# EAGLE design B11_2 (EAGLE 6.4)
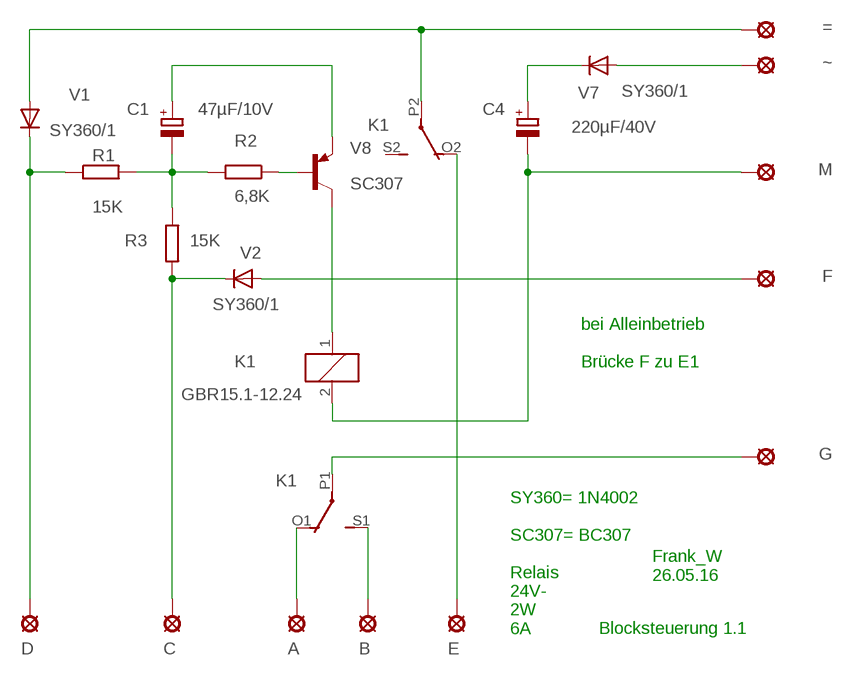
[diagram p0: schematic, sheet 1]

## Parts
=  LSP10  [LSP10]
A  LSP10  [LSP10]
B  LSP10  [LSP10]
C  LSP10  [LSP10]
C1  47µF/10V  CPOL-EUE5-5  [E5-5]
C4  220µF/40V  CPOL-EUE22-9AXIAL  [E22-9]
D  LSP10  [LSP10]
E  LSP10  [LSP10]
F  LSP10  [LSP10]
G  LSP10  [LSP10]
K1  GBR15.1-12.24  4052  [F4052]
M  LSP10  [LSP10]
R1  15K  R-EU_0207/12  [0207/12]
R2  6,8K  R-EU_0207/12  [0207/12]
R3  15K  R-EU_0207/12  [0207/12]
V1  SY360/1  1N4004  [DO41-10]
V2  SY360/1  1N4004  [DO41-10]
V7  SY360/1  1N4004  [DO41-10]
V8  SC307  BC307  [TO92]
~  LSP10  [LSP10]

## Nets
N$1: F.MP V2.A
N$2: C4.- K1.2 M.MP
N$3: =.MP K1.P2(3:P) V1.A
N$4: C4.+ V7.C
N$5: K1.1 V8.3(C)
N$6: C1.- R1.2 R2.2 R3.1
N$7: A.MP K1.O1(2:O)
N$8: R2.1 V8.2(B)
N$9: D.MP R1.1 V1.C
N$10: C.MP R3.2 V2.C
N$12: B.MP K1.S1(2:S)
N$13: V7.A ~.MP
N$14: E.MP K1.O2(3:O)
N$25: G.MP K1.P1(2:P)
N$42: C1.+ V8.1(E)
Unconnected: K1.S2(3:S)

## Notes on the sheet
- bei Alleinbetrieb
  
  Brücke F zu E1
- Frank_W 
  26.05.16
- SY360= 1N4002 
  
  SC307= BC307
  
  Relais 
  24V-
  2W
  6A
- Blocksteuerung 1.1

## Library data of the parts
= A B C D E F G M ~ = solpad:LSP10: SOLDER PAD
C1 C4 = rcl:CPOL-EU: POLARIZED CAPACITOR, European symbol
K1 = relay:4052: RELAY 2 x switch, Finder; OC_FARNELL: unknown; OC_NEWARK: unknown
R1-R3 = rcl:R-EU_: RESISTOR, European symbol
V1 V2 V7 = diode:1N4004: DIODE
V8 = transistor-pnp:BC307: PNP Transistor

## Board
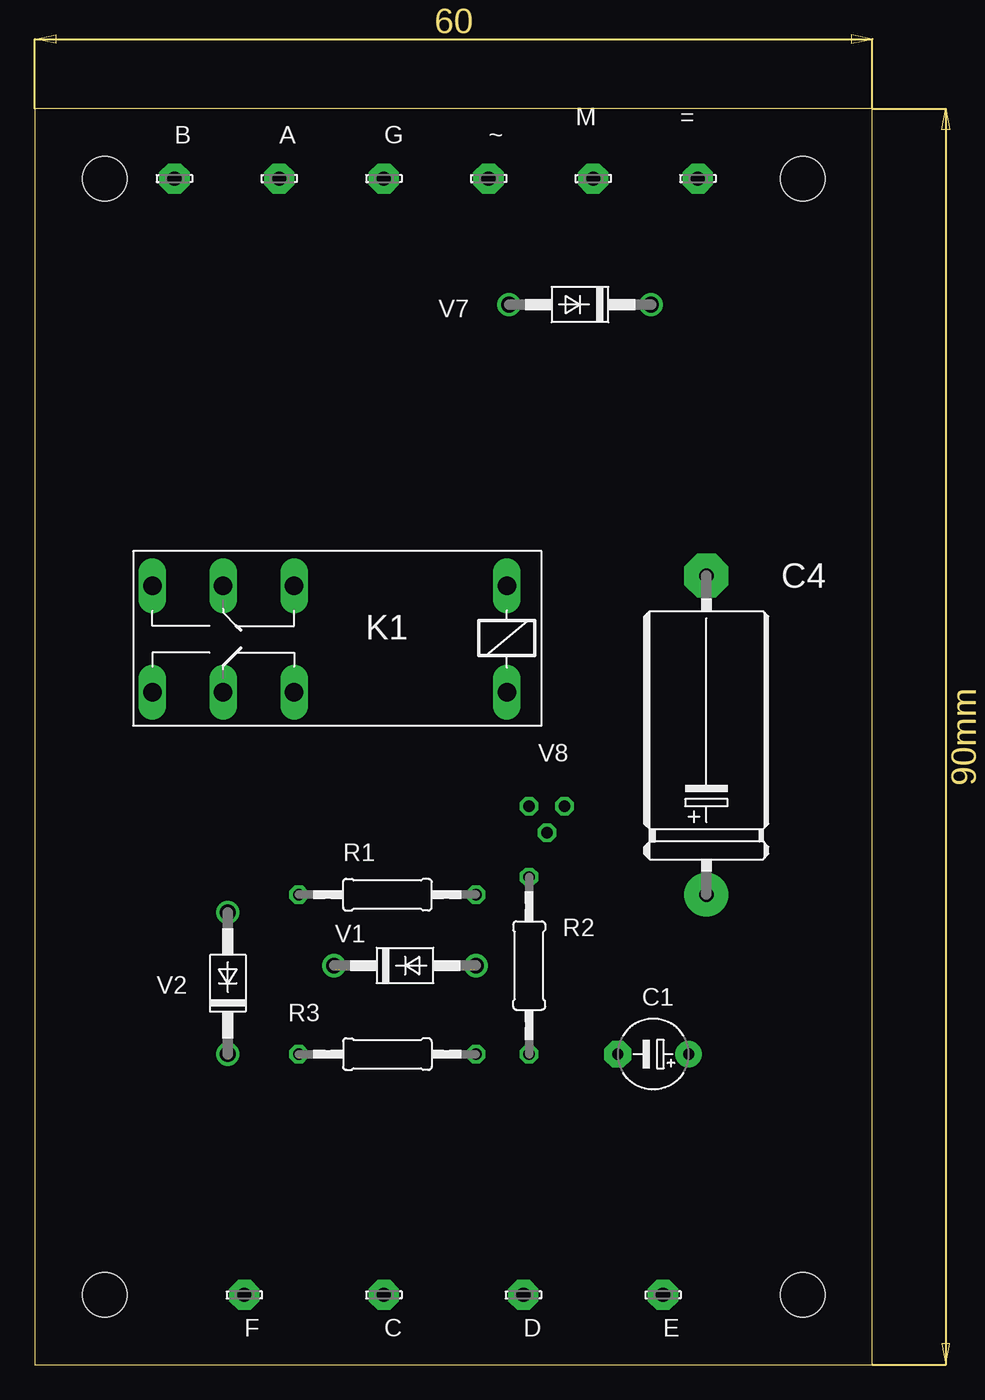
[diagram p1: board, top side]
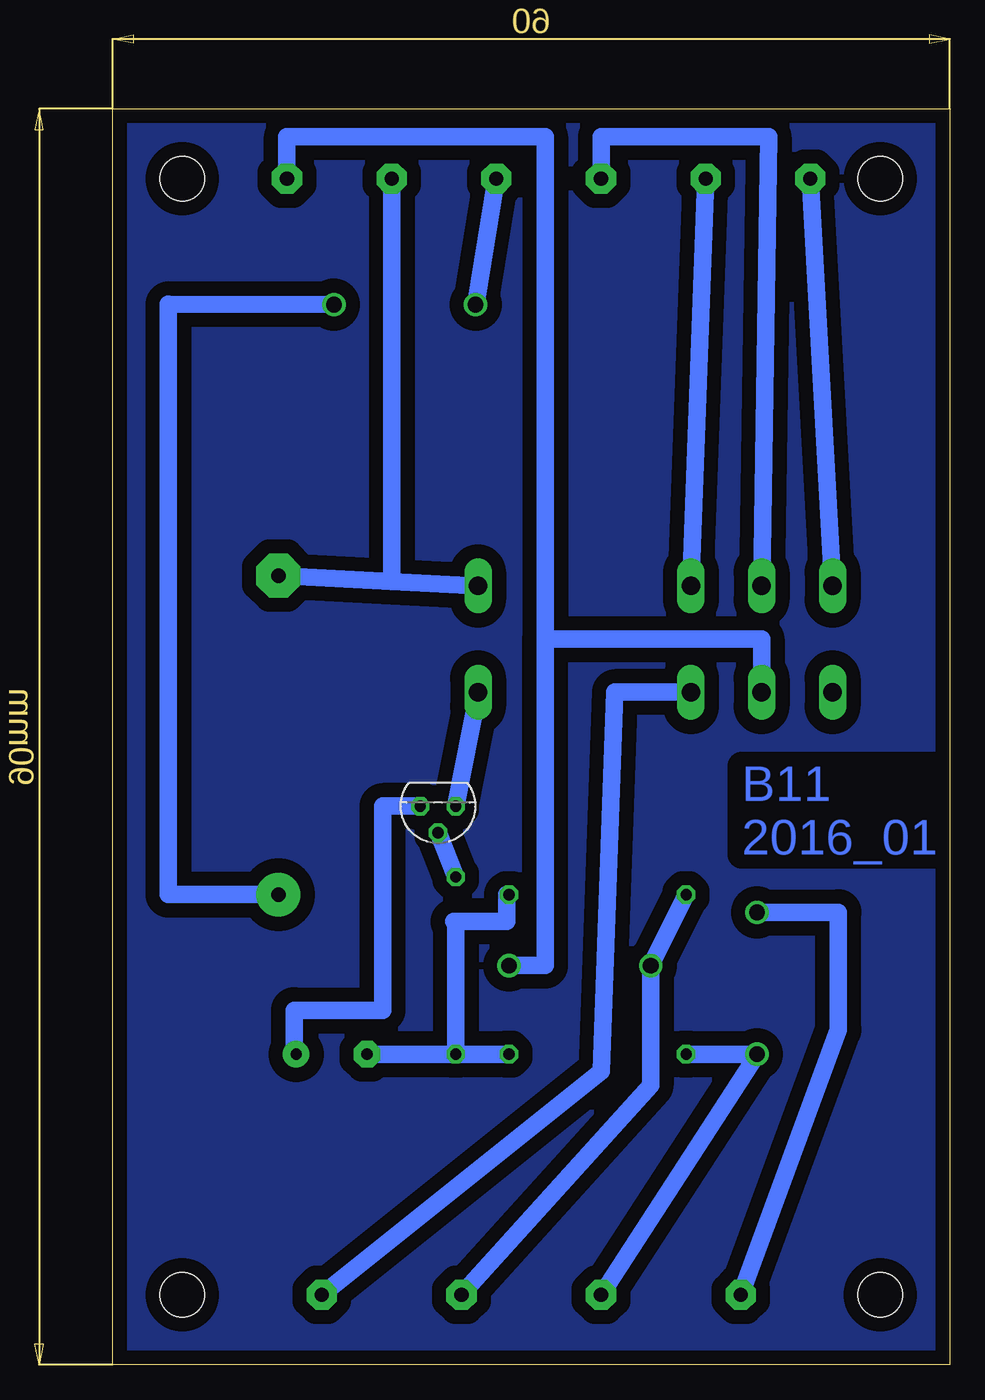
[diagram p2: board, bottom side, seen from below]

Size 65.56 x 95.3 mm. Coordinates in mm from the lower left corner, seen from the top.
Outline: 0,90 0,0 60,0 60,90 0,90
Copper layers (1*16): Top 0.035mm / dielectric 1.5mm / Bottom 0.035mm
Design rules "default *": minimum track width 20mil, minimum drill 24mil, track to track 8mil, track to pad 8mil, pad to pad 8mil, via to via 8mil, smd to smd 8mil, copper to edge 40mil, drill to drill 8mil, minimum pad ring 10mil, minimum via ring 8mil, stop-mask expansion 4mil, vias tented up to drill 0mil, thermal gap 20mil
Holes 3.2 mm at 55,5 5,85 5,5 55,85

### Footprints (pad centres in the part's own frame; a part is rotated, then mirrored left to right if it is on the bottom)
LSP10 = drill 1.016 pad 2.159 octagon: MP 0,0
E5-5 = drill 0.813 pad 1.905: + -2.54,0 | drill 0.813 pad 1.905 octagon: - 2.54,0
E22-9 = drill 1.016 pad 3.15: + -11.43,0 | drill 1.016 pad 3.15 octagon: - 11.43,0
F4052 = drill 1.321 long: 1 -3.81,3.81; 2 -3.81,-3.81; O1 11.43,-3.81; O2 11.43,3.81; P1 16.51,-3.81; P2 16.51,3.81; S1 21.59,-3.81; S2 21.59,3.81
0207/12 = drill 0.813 octagon: 1 -6.35,0; 2 6.35,0
DO41-10 = drill 1.118: A 5.08,0; C -5.08,0
TO92 = drill 0.813 octagon: 1 1.27,0; 2 0,1.905; 3 -1.27,0

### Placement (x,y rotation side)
=  47.5,85 0 top
A  17.5,85 0 top
B  10,85 0 top
C  25,5 0 top
C1  44.3,22.25 180 top
C4  48.11,45.11 90 top
D  35,5 0 top
E  45,5 0 top
F  15,5 0 top
G  25,85 0 top
K1  30,52 180 top
M  40,85 0 top
R1  25.25,33.68 0 top
R2  35.41,28.6 270 top
R3  25.25,22.25 180 top
V1  26.52,28.6 0 top
V2  13.82,27.33 90 top
V7  39.06,75.97 180 top
V8  36.68,40.03 180 bottom
~  32.5,85 0 top

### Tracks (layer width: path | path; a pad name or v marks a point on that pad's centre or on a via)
N$1
  Bottom 1.27: F.MP 8,24 8,32.41 V2.A
N$2
  Bottom 1.27: C4.- 39.99,56.13 | 39.99,56.13 K1.2 | M.MP 39.99,56.13
N$3
  Bottom 1.27: =.MP 47.5,88 29,88 29,52 | 29,52 13.49,52 K1.P2 | V1.A 29,28.6 29,52
N$4
  Bottom 1.27: V7.C 56,76 56,33.68 C4.+
N$5
  Bottom 1.27: V8.3 K1.1
N$6
  Bottom 1.27: R3.1 R2.2 | R2.2 C1.- | R1.2 31.75,33.68 31.75,31.75 35.41,31.75 | 35.56,31.75 35.41,31.75 | 35.41,31.75 R2.2
N$7
  Bottom 1.27: K1.O1 A.MP
N$8
  Bottom 1.27: R2.1 V8.2
N$9
  Bottom 1.27: R1.1 V1.C 21.44,20 D.MP
N$10
  Bottom 1.27: C.MP V2.C R3.2
N$11
  pour Bottom (isolate 1.016): 0,90 60,90 60,0 0,0
N$12
  Bottom 1.27: K1.S1 B.MP
N$13
  Bottom 1.27: V7.A ~.MP
N$14
  Bottom 1.27: K1.O2 24,48.19 25,21 E.MP
N$25
  Bottom 1.27: G.MP 25,88 13,88 K1.P1
N$42
  Bottom 1.27: C1.+ 46.99,22.25 46.99,25.4 40.64,25.4 40.64,40.03 V8.1

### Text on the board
Bottom: B11 / 2016_01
